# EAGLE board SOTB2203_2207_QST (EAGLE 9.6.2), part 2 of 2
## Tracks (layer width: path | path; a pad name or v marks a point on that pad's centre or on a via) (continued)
PKG1/FR_CO_CH4/FR_CI_CH3  (via drill 0.3) (continued)
  Top 0.152: PKG1.71 58.83,77.28 59.24,76.87 66.99,76.87 73.13,83.01 73.13,112.99 66.99,119.13 65.01,119.13 v64.68,119.46 | v64.71,118.25 64.67,118.22 PKG1.121
  Bottom 0.152: v64.71,118.25 64.68,118.27 v64.68,119.46
PKG1/FR_SO  (via drill 0.3)
  Top 0.152: PKG1.113 v71.4,106.12 v71.41,106.12 | v73.74,106.12 74.34,106.72 74.34,107.66 73.69,108.31 73.69,113.22 67.22,119.69 65.82,119.69 65.16,120.34 64.31,120.34 64.22,120.25 36.53,120.25 29.75,113.47 29.75,98.87 29.1,98.22 29.1,97.48 29.47,97.11 29.47,92.98 28.82,92.33 28.82,91.59 29.19,91.22 29.19,65.39 29.1,65.3 29.1,63.27 29.72,62.65 29.72,35.38 37.02,28.07 66.93,28.07 67.26,27.75 v67.26,27.19 | v67.26,25.14 67.38,25.02 67.38,18.97 68.5,17.85 CN1.A19 69.93,16.57 69.93,6.24 CN5.A19
  Bottom 0.152: v71.41,106.12 v73.74,106.12 | v67.26,27.19 v67.26,25.14
PKG1/FR_SO_CH1/FR_SI_CH2  (via drill 0.3)
  Top 0.152: PKG1.153 43.88,118.16 43.18,118.85 37.12,118.85 31.15,112.88 31.15,97.33 30.59,96.77 30.59,91.59 30.03,91.03 30.03,82.66 36.66,76.03 40.29,76.03 v40.62,75.7 | PKG1.43 40.62,78.43 v40.66,78.4
  Bottom 0.152: v40.66,78.4 40.62,78.36 v40.62,75.7
PKG1/FR_SO_CH2/FR_SI_CH3  (via drill 0.3)
  Top 0.152: v74.3,86.62 73.97,86.29 73.97,82.66 67.34,76.03 58.89,76.03 58.34,76.59 53.25,76.59 52.69,77.15 37.12,77.15 31.15,83.12 31.15,89.32 31.7,89.88 PKG1.33 | PKG1.83 71.42,86.62 v71.82,87.02
  Bottom 0.152: v74.3,86.62 74.29,86.63 72.25,86.63 71.86,87.02 v71.82,87.02
PKG1/FR_SO_CH3/FR_SI_CH4  (via drill 0.3)
  Top 0.152: PKG1.73 60.12,77.55 60.52,77.15 66.88,77.15 72.85,83.12 72.85,112.88 66.88,118.85 63.45,118.85 v63.37,118.93 | PKG1.123 63.38,117.54 v63.34,117.57
  Bottom 0.152: v63.37,118.93 63.37,117.59 v63.34,117.57
PKG1/TFT_CO  (via drill 0.3)
  Top 0.152: PKG1.149 46.48,117.94 v46.81,118.28 | v46.81,120.85 46.48,120.53 36.41,120.53 29.47,113.59 29.47,98.98 28.82,98.33 28.82,97.37 29.19,97 29.19,93.09 28.54,92.44 28.54,91.48 28.91,91.11 28.91,65.51 28.82,65.41 28.82,63.15 29.44,62.53 29.44,35.26 36.91,27.79 65.66,27.79 65.99,27.47 v65.99,27.19 | v65.99,25.14 66.01,25.12 66.01,23.03 CN1.C20
  Route15 0.152: CN1.C20 64.81,21.63 64.81,11.34 CN5.C20
  Bottom 0.152: v46.81,118.28 v46.81,120.85 | v65.99,27.19 v65.99,25.14
PKG1/TFT_CO_CH2/TFT_CI_CH1  (via drill 0.3)
  Top 0.152: PKG1.29 32.23,92.47 31.75,92.96 v31.75,95.12 | PKG1.142 51.02,118.56 50.41,119.16 44.73,119.16 44.2,119.69 36.76,119.69 30.31,113.24 30.31,98.18 v29.98,97.85
  Bottom 0.152: v31.75,95.12 31.75,97.52 31.42,97.85 v29.98,97.85
PKG1/TFT_CO_CH3/TFT_CI_CH2  (via drill 0.3)
  Top 0.152: PKG1.22 31.24,97.03 30.87,96.65 30.87,91.48 30.31,90.92 30.31,82.78 36.78,76.31 51.63,76.31 52.35,76.31 52.9,75.75 56.82,75.75 v57.15,75.42 | PKG1.69 57.52,78.11 57.19,77.78 v57.19,77.75
  Bottom 0.152: v57.19,77.75 57.19,75.46 v57.15,75.42
PKG1/TFT_CO_CH4/TFT_CI_CH3  (via drill 0.3)
  Top 0.152: PKG1.62 52.98,77.26 53.37,76.87 58.45,76.87 59.01,76.31 67.22,76.31 73.69,82.78 73.69,102.92 v74.02,103.25 | PKG1.109 71.41,103.53 v71.69,103.25
  Bottom 0.152: v74.02,103.25 v71.69,103.25
PKG1/TFT_SO  (via drill 0.3)
  Top 0.152: PKG1.104 71.97,100.28 72.29,100.59 72.29,108 72.13,108.16 v71.97,108.16 | v73.74,107.41 73.41,107.74 73.41,113.11 67.11,119.41 65.7,119.41 65.05,120.06 64.43,120.06 64.34,119.97 36.65,119.97 30.03,113.35 30.03,98.75 29.38,98.1 29.38,97.6 29.75,97.23 29.75,92.86 29.1,92.21 29.1,91.71 29.47,91.34 29.47,65.28 29.38,65.18 29.38,63.38 30,62.77 30,35.49 37.14,28.35 68.22,28.35 68.57,28.01 v68.57,27.19 | CN1.C19 68.57,23.01 v68.57,25.14
  Route15 0.152: CN1.C19 68.34,22.93 67.4,21.99 67.4,11.29 CN5.C19
  Bottom 0.152: v71.97,108.16 71.97,107.56 72.12,107.41 v73.74,107.41 | v68.57,27.19 v68.57,25.14
PKG1/TFT_SO_CH1/TFT_SI_CH2  (via drill 0.3)
  Top 0.152: PKG1.30 31.8,91.83 v31.75,91.78 | v29.7,91.96 30.03,92.29 30.03,97 30.59,97.56 30.59,113.12 36.88,119.41 44.08,119.41 44.61,118.88 49.3,118.88 49.73,118.45 PKG1.144 | v29.7,91.96
  Bottom 0.152: v29.7,91.96 31.57,91.96 v31.75,91.78
PKG1/TFT_SO_CH2/TFT_SI_CH3  (via drill 0.3)
  Top 0.152: PKG1.24 31.47,95.72 31.15,95.4 31.15,91.36 31.13,91.35 31.12,91.33 30.59,90.8 30.59,82.89 36.89,76.59 52.46,76.59 53.02,76.03 57.74,76.03 57.97,75.8 v57.97,75.7 | PKG1.70 v58.17,77.76 v58.17,77.75
  Bottom 0.152: v58.17,77.75 57.97,77.55 v57.97,75.7
PKG1/TFT_SO_CH3/TFT_SI_CH4  (via drill 0.3)
  Top 0.152: PKG1.64 54.27,77.5 54.63,77.15 58.57,77.15 59.13,76.59 67.11,76.59 73.41,82.89 73.41,103.85 v73.74,104.18 | v71.69,104.18 PKG1.110
  Bottom 0.152: v73.74,104.18 v71.69,104.18
PKG4/A_SOUT_CH1  (via drill 0.3)
  Top 0.152: PKG4.15 114.18,48.39 v117.54,48.39 | CN7.A20 85.16,143.77 85.16,133.42 CN3.A20 82.64,130.9 82.64,123.26 83.97,121.93 114.16,121.93 122.03,114.06 122.03,72.84 122.48,72.39 122.48,59.47 123.14,58.82 123.14,55.84 122.48,55.19 122.48,48.55 v122.31,48.38
  Bottom 0.152: v117.54,48.39 122.3,48.39 v122.31,48.38
PKG4/A_SOUT_CH2  (via drill 0.3)
  Top 0.152: v101.77,71.82 101.58,71.62 PKG4.55 | v101.78,74.3 102.11,73.97 108.2,73.97 109.13,74.9 110.15,74.9 110.43,75.18 117.22,75.18 117.36,75.04 117.36,72.73 v118.81,71.29 | CN7.A19 82.62,143.77 82.62,133.42 CN3.A19 80.12,130.92 80.12,122.52 81.27,121.37 113.93,121.37 121.47,113.83 v121.47,72.15
  Bottom 0.152: v101.77,71.82 101.77,74.29 v101.78,74.3 | v118.81,71.29 120.61,71.29 v121.47,72.15
PKG4/A_SOUT_CH3  (via drill 0.3)
  Top 0.152: v75.7,53.53 75.7,55.57 76.03,55.89 76.03,62.02 74.82,63.23 74.82,64.93 75.47,65.58 75.47,82.3 75.74,82.57 75.74,86.82 75.46,87.1 75.46,107.84 75.64,108.02 75.64,112.47 72.46,115.64 72.46,130.88 CN3.A16 75,133.42 75,143.77 CN7.A16 | v78.18,55.8 78.96,55.8 79.19,55.58 PKG4.95
  Bottom 0.152: v75.7,53.53 75.7,53.47 76.02,53.16 76.28,53.16 77.15,54.03 77.15,54.76 v78.18,55.8
PKG4/A_SOUT_CH4  (via drill 0.3)
  Top 0.152: PKG4.135 94.39,35.82 v94.39,32.43 | CN3.C19 81.35,122.88 82.24,121.99 82.3,121.93 82.58,121.65 114.05,121.65 121.75,113.94 121.75,72.73 122.21,72.27 122.21,59.36 122.86,58.71 122.86,55.95 122.21,55.3 122.21,52.07 121.65,51.52 121.65,42.79 122.86,41.58 122.86,38.26 122.21,37.61 122.21,35.72 114.28,27.79 105.86,27.79 105.13,27.06 104.39,27.06 104.07,27.39 102.14,27.39 101.49,28.04 95.79,28.04 95.44,27.69 v94.65,27.69
  Route15 0.152: CN7.C19 82.62,138.69 82.62,128.34 CN3.C19
  Bottom 0.152: v94.39,32.43 94.39,27.94 v94.65,27.69
PKG4/FR_CO  (via drill 0.3)
  Top 0.152: PKG4.1 v118.24,39.33 v118.25,39.32 | v120.3,39.32 119.97,38.99 119.97,36.65 113.35,30.03 105.69,30.03 105.16,30.56 87.11,30.56 86.49,29.94 85.05,29.94 84.4,30.59 78.05,30.59 77.4,29.94 v77.4,27.19 | v77.4,25.14 77.55,24.99 77.55,19.25 78.81,17.99 CN1.A15 80.09,16.57 80.09,6.42 80.09,6.24 CN5.A15
  Bottom 0.152: v118.25,39.32 v120.3,39.32 | v77.4,27.19 v77.4,25.14
PKG4/FR_CO_CH2/FR_CI_CH1  (via drill 0.3)
  Top 0.152: PKG4.151 104.83,32.08 106.03,30.87 113.01,30.87 119.13,36.99 119.13,52.56 119.69,53.12 119.69,58.29 120.25,58.85 120.25,67.45 113.45,74.25 111.01,74.25 v110.68,74.58 | PKG4.41 v110.67,72.24 v110.68,72.25
  Bottom 0.152: v110.68,72.25 v110.68,74.58
PKG4/FR_CO_CH3/FR_CI_CH2  (via drill 0.3)
  Top 0.152: PKG4.81 v77.76,64.67 v77.75,64.68 | v75.42,64.68 75.75,65.01 75.75,67.45 82.55,74.25 91.22,74.25 91.78,73.69 96.86,73.69 97.42,73.13 98,73.13 98.08,73.13 112.99,73.13 119.13,66.99 119.13,59.31 118.65,58.83 PKG4.31
  Bottom 0.152: v77.75,64.68 v75.42,64.68
PKG4/FR_CO_CH4/FR_CI_CH3  (via drill 0.3)
  Top 0.152: PKG4.121 85.33,32.05 85.29,32.01 v85.29,31.75 | PKG4.71 91.17,72.72 90.76,73.13 83.01,73.13 76.87,66.99 76.87,37.01 83.01,30.87 84.97,30.87 v85.3,30.54
  Bottom 0.152: v85.29,31.75 v85.3,31.75 v85.3,30.54
PKG4/FR_SO  (via drill 0.3)
  Top 0.152: PKG4.113 v78.6,43.88 v78.59,43.87 | v76.26,43.87 76.26,43.02 75.66,42.41 75.66,41.91 75.75,41.82 75.75,27.96 v74.98,27.19 | v74.98,25.14 74.98,19.21 76.27,17.92 CN1.A16 77.53,16.59 77.53,6.42 77.53,6.22 CN5.A16
  Bottom 0.152: v78.59,43.87 v76.26,43.87 | v74.98,27.19 v74.98,25.14
PKG4/FR_SO_CH1/FR_SI_CH2  (via drill 0.3)
  Top 0.152: PKG4.153 106.12,31.84 106.82,31.15 112.88,31.15 118.85,37.12 118.85,52.67 119.41,53.23 119.41,58.41 119.97,58.97 119.97,67.34 113.34,73.97 109.71,73.97 v109.38,74.3 | PKG4.43 109.38,71.57 v109.13,71.82
  Bottom 0.152: v109.13,71.82 109.38,72.06 v109.38,74.3
PKG4/FR_SO_CH2/FR_SI_CH3  (via drill 0.3)
  Top 0.152: v75.7,63.38 76.03,63.71 76.03,67.34 82.66,73.97 91.11,73.97 91.66,73.41 96.75,73.41 97.31,72.85 112.88,72.85 118.85,66.88 118.85,60.68 118.3,60.12 PKG4.33 | PKG4.83 78.58,63.38 v78.18,62.98
  Bottom 0.152: v75.7,63.38 75.71,63.37 77.75,63.37 78.14,62.98 v78.18,62.98
PKG4/FR_SO_CH3/FR_SI_CH4  (via drill 0.3)
  Top 0.152: PKG4.73 89.88,72.45 89.48,72.85 83.12,72.85 77.15,66.88 77.15,37.12 83.12,31.15 86.69,31.15 v86.77,31.07 | PKG4.123 86.62,32.46 v86.66,32.43
  Bottom 0.152: v86.66,32.43 86.66,31.18 v86.77,31.07
PKG4/TFT_CO  (via drill 0.3)
  Top 0.152: PKG4.149 103.53,31.88 103.36,31.72 v103.2,31.72 | v103.2,29.95 102.87,30.28 87.23,30.28 86.61,29.66 84.93,29.66 84.28,30.31 79.18,30.31 78.71,29.84 v78.71,27.19 | v78.71,25.14 78.78,25.07 78.78,22.96 CN1.C15
  Route15 0.152: CN1.C15 77.55,21.67 77.55,11.5 77.55,11.3 CN5.C15
  Bottom 0.152: v103.2,31.72 v103.2,29.95 | v78.71,27.19 v78.71,25.14
PKG4/TFT_CO_CH2/TFT_CI_CH1  (via drill 0.3)
  Top 0.152: PKG4.29 117.77,57.52 118.06,57.23 v118.25,57.23 | v120.58,56.9 120.25,56.57 120.25,52.88 119.69,52.33 119.69,36.76 113.24,30.31 105.8,30.31 105.27,30.84 99.59,30.84 98.97,31.45 PKG4.142
  Bottom 0.152: v118.25,57.23 118.58,56.9 v120.58,56.9
PKG4/TFT_CO_CH3/TFT_CI_CH2  (via drill 0.3)
  Top 0.152: PKG4.22 118.76,52.98 119.13,53.35 119.13,58.52 119.69,59.08 119.69,67.22 113.22,73.69 97.65,73.69 97.1,74.25 92.51,74.25 v92.18,74.58 | PKG4.69 92.47,71.89 92.81,72.22 v92.81,72.25
  Bottom 0.152: v92.18,74.58 92.81,73.95 v92.81,72.25
PKG4/TFT_CO_CH4/TFT_CI_CH3  (via drill 0.3)
  Top 0.152: PKG4.62 97.03,72.74 96.63,73.13 91.55,73.13 90.99,73.69 82.78,73.69 76.31,67.22 76.31,47.08 v75.98,46.75 | PKG4.109 78.59,46.48 v78.31,46.75
  Bottom 0.152: v75.98,46.75 v78.31,46.75
PKG4/TFT_SO  (via drill 0.3)
  Top 0.152: PKG4.104 78.03,49.73 77.71,49.4 77.71,42.49 v78.03,42.16 | v76.26,42.16 76.59,41.83 76.59,27.61 v76.17,27.19 | CN1.C16 76.17,23.03 v76.17,25.14
  Route15 0.152: CN1.C16 75.01,21.67 75.01,11.5 75.01,11.3 CN5.C16
  Bottom 0.152: v78.03,42.16 v76.26,42.16 | v76.17,27.19 v76.17,25.14
PKG4/TFT_SO_CH1/TFT_SI_CH2  (via drill 0.3)
  Top 0.152: PKG4.30 118.2,58.17 v118.25,58.22 | v120.3,58.04 119.97,57.71 119.97,53 119.41,52.44 119.41,36.88 113.12,30.59 105.92,30.59 105.39,31.12 100.7,31.12 100.28,31.55 PKG4.144
  Bottom 0.152: v120.3,58.04 118.43,58.04 v118.25,58.22
PKG4/TFT_SO_CH2/TFT_SI_CH3  (via drill 0.3)
  Top 0.152: PKG4.24 118.53,54.27 118.85,54.6 118.85,58.64 118.87,58.65 118.88,58.67 119.41,59.2 119.41,67.11 113.11,73.41 97.54,73.41 96.98,73.97 91.89,73.97 91.01,74.86 v90.95,74.86 | PKG4.70 v91.83,72.24 v91.83,72.25
  Bottom 0.152: v91.83,72.25 91.83,73.98 v90.95,74.86
PKG4/TFT_SO_CH3/TFT_SI_CH4  (via drill 0.3)
  Top 0.152: PKG4.64 95.72,72.5 95.37,72.85 91.43,72.85 90.87,73.41 82.89,73.41 76.59,67.11 76.59,46.15 v76.26,45.82 | v78.31,45.82 PKG4.110
  Bottom 0.152: v76.26,45.82 v78.31,45.82
TFT_CI  (via drill 0.3, 0.35)
  Top 0.152: PKG4.102 77.81,51.02 77.43,50.64 77.43,39.65 77.82,39.25 79.28,39.25 84.3,34.22 v84.62,34.22 | PKG1.102 72.19,98.97 72.57,99.36 72.57,110.28 72.14,110.71 70.63,110.71 65.56,115.78 v65.38,115.78 | v65.38,121.23 65.05,120.9 64.08,120.9 63.99,120.81 48.2,120.81 47.27,121.74 46.44,121.74 45.79,121.09 36.18,121.09 28.91,113.82 28.91,112.02 27.98,111.09 27.98,110.3 28.63,109.65 28.63,99.33 27.98,98.68 27.98,97.02 28.35,96.65 28.35,93.44 27.7,92.79 27.7,91.13 28.07,90.76 28.07,78.33 27.42,77.68 27.42,76.53 v27.75,76.2 28.07,75.87 28.07,67.04 27.42,66.39 27.42,65.89 27.66,65.65 v27.66,65.38 27.98,65.05 27.98,62.81 28.6,62.19 28.6,34.91 36.56,26.96 63.67,26.96 64.32,26.3 84.11,26.3 84.76,25.65 85.37,25.65 v85.69,25.98 86.02,26.3 86.02,27.88 86.4,28.26 87.19,28.26 87.81,28.88 101.84,28.88 102.49,28.23 103.91,28.23 104.32,28.63 113.93,28.63 121.37,36.07 121.37,37.95 122.02,38.61 122.02,40.03 121.09,40.97 121.09,51.75 121.65,52.31 121.65,55.53 122.3,56.19 122.3,58.47 121.65,59.13 121.65,68.03 120.53,69.15 120.53,76.3 119.55,77.28 v119.55,78.89 | CN4.C17 23,76.2 v25.65,76.2 | v59.4,34.3 58.9,34.3 58.48,34.72 38.88,34.72 34.72,38.88 34.72,44.28 v34.3,44.7 34.3,44.9 34.72,45.32 34.72,65.72 v35,66 v37.7,68.7 38.28,69.28 65.82,69.28 69.5,65.6 69.5,61.5 67.5,59.5 JP2.3 | JP14.3 113.5,105.5 115.5,107.5 115.5,111.6 111.82,115.28 84.28,115.28 v83.7,114.7 80.72,111.72 80.72,91.32 80.3,90.9 v80.3,90.3 80.3,89.9 80.72,89.48 80.72,84.88 84.88,80.72 104.48,80.72 104.9,80.3 v105.4,80.3 106.05,79.65 116.95,79.65 v117.6,79
  Route2 0.152: v27.66,65.38 34,65.38 34.62,66 v35,66
  Route15 0.152: CN4.C17 21.69,77.51 11.28,77.51 CN8.C17
  Bottom 0.152: v65.38,115.78 v65.38,121.23 | v27.75,76.2 v25.65,76.2 | v84.62,34.22 84.62,29.09 85.69,28.01 v85.69,25.98 | v59.4,34.3 59.5,34.4 JP4.3 | v34.3,44.7 34.5,44.5 JP6.3 | v37.7,68.7 43.8,68.7 44.5,68 JP8.3 | v105.4,80.3 105.5,80.4 JP16.3 | v80.3,90.3 80.5,90.5 JP10.3 | v83.7,114.7 89.8,114.7 90.5,114 JP12.3 | v117.6,79 119.44,79 v119.55,78.89
TFT_SI  (via drill 0.3, 0.35)
  Top 0.152: PKG1.150 45.83,118.23 v45.78,118.28 | v104.3,31.72 104.17,31.84 PKG4.150 | v45.54,121.69 45.22,121.37 36.07,121.37 28.63,113.93 28.63,112.13 27.7,111.2 27.7,110.19 28.35,109.54 28.35,99.45 27.7,98.8 27.7,96.91 28.07,96.53 28.07,93.56 27.42,92.91 27.42,91.02 27.79,90.64 27.79,78.45 27.14,77.8 27.14,75.34 v27.47,75.01 27.79,74.68 27.79,67.16 27.05,66.41 27.05,65.13 27.7,64.48 27.7,62.69 28.32,62.07 28.32,46.32 27.94,45.94 v27.94,45.39 28.32,45.01 28.32,34.8 36.44,26.68 36.5,26.68 63.55,26.68 64.2,26.02 83.99,26.02 84.65,25.37 85.95,25.37 86.3,25.73 86.3,27.77 86.51,27.98 87.3,27.98 87.92,28.6 101.72,28.6 102.37,27.95 v104.76,27.95 105.16,28.35 114.05,28.35 121.65,35.95 121.65,37.84 122.3,38.49 122.3,40.15 121.37,41.08 121.37,51.63 121.93,52.19 121.93,55.42 122.58,56.07 122.58,58.59 121.93,59.24 121.93,68.15 120.81,69.27 120.81,76.42 120.2,77.03 v120.2,79.8 | v25.65,75 18.84,75 17.85,74.01 CN4.A16 16.6,72.48 6.21,72.48 CN8.A16 | JP7.1 35.08,54.42 | 35.08,54.42 35,54.5 | 35,54.5 35,65 39,69 54,69 54.42,68.58 JP1.1 | 35,54.5 35,54.34 | 35,54.34 35,47.1 | 35,47.1 35,47 | 35,47 35,46.9 | 35,46.9 35,39 39,35 49.33,35 | 49.58,35.08 49.58,35.25 | JP5.1 49.58,35.25 | 49.33,35 49.83,35 | 49.83,35 65.5,35 69,38.5 69,49 68.42,49.58 JP3.1 | 35,54.34 35.08,54.42 | v35.7,46.2 35.7,46.8 35.5,47 35.1,47 | 35,47 35.1,47 | 35,47.1 35.1,47 | 35.1,47 35,46.9 | JP11.1 81.08,100.42 | 81.08,100.42 81,100.5 | 81,100.5 81,111 85,115 100,115 100.42,114.58 JP13.1 | 81,100.5 81,100.34 | 81,100.34 81,85 85,81 95.41,81 | 95.58,81.08 95.58,81.17 | 95.58,81.17 JP9.1 | 95.41,81 95.75,81 | 95.75,81 v110.2,81 111.5,81 115,84.5 115,95 114.42,95.58 JP15.1
  Top 0.152: 81,100.34 81.08,100.42 | 49.58,35.25 49.33,35 | 95.75,81 95.58,81.17 | 95.58,81.17 95.41,81 | 49.58,35.25 49.83,35
  Bottom 0.152: v45.54,121.69 45.78,121.45 v45.78,118.28 | v104.76,27.95 104.76,31.26 v104.3,31.72 | v27.47,75.01 v25.66,75.01 v25.65,75 | v27.94,45.39 34.9,45.39 v35.7,46.2 | v110.2,81 111,80.2 119.8,80.2 v120.2,79.8
VBN  (via drill 0.3, 0.35, 0.8, 1.27)
  Top 0.305: PKG1.158 40.62,111.97 v40.5,111.84 | PKG1.118 66.03,109.38 v65.89,109.51 | PKG1.38 37.95,86.62 v38.07,86.5 | PKG1.78 63.38,83.89 v63.5,84.01 | PKG4.78 86.62,66.08 v86.5,65.95 | PKG4.38 112.13,63.38 v112.01,63.5 | PKG4.158 109.38,37.97 v109.47,38.06 | PKG4.118 83.88,40.62 v84,40.5
  Top 0.508: CN4.C21 21.66,87.7 11.31,87.7 CN8.C21
  Route2 0.305: v95.29,39.46 95.29,37.85 95.89,37.25 108.66,37.25 v109.47,38.06 | v112.01,63.5 112.51,63.5 112.85,63.84 112.85,77.24 111.91,78.17 v109.92,78.17 | v65.7,77.75 63.86,77.75 63.5,78.11 v63.5,84.01 | v38.3,77.75 38.3,75.04 38.71,74.63 39.33,74.63 44.67,69.28 47.7,69.28 49.58,67.4 JP8.5 | v49.39,106.27 51.4,106.27 52.42,107.29 64.65,107.29 65.13,107.77 65.13,109.13 65.51,109.51 v65.89,109.51
  Route2 1.016: v71.47,78.01 72.84,76.64 72.84,70.23 v73.62,69.45
  Bottom 0.305: v40.5,111.84 C20.1 | v65.89,109.51 C15.1 | v38.07,86.5 C5.1 | v63.5,84.01 C10.1 | v86.5,65.95 C70.1 | v112.01,63.5 C65.1 | v109.47,38.06 109.5,38.09 C80.1 | v84,40.5 C75.1 | JP8.5 48.5,65.42 C35.1 49.38,60 v55,60 | JP2.5 65.42,55.5 v62.5,55.5 C30.1 | JP4.5 55.5,38.58 v55.5,41.5 C25.1 | JP6.5 38.58,48.5 C40.1 44.62,50 v56,50 | JP10.5 84.6,94.48 89.11,94.48 C50.1 90.62,96 v102,96 | JP12.5 94.5,111.42 C45.1 95.38,106 v101,106 | JP14.5 111.42,101.5 v108.5,101.5 C60.1 | JP16.5 101.5,84.58 v101.5,87.5 C55.1
  Bottom 1.27: v32.5,77.5 32.5,82.37 31.25,83.62 29.57,83.62 28.9,84.29 U$8.+ 22.95,86.41 CN4.C21
  other vias: 83,67 84,68 82,66
  pour Route15: 55,70 54,69 54,35 55,34 65,34 70,39 70,65 65,70
  pour Route15: 32,79 111,79 111,77 110,76 32,76 31,77 31,78
  pour Route15: 39,116 34,111 34,80 33,79 51,79 50,80 50,115 49,116
  pour Route15: 85,70 80,65 80,39 85,34 95,34 96,35 96,69 95,70
  pour Route15: 101,116 100,115 100,80 99,79 111,79 116,84 116,111 111,116
  pour Route15: 65,70 65,65 85,65 85,70
VBP  (via drill 0.3, 0.35, 0.8, 1.27)
  Top 0.305: PKG1.157 41.27,112.03 41.44,111.86 v42,111.86 | PKG1.117 66.14,108.72 65.92,108.51 v65.92,108 | PKG1.37 37.91,87.28 38.04,87.41 v38.04,88 | v61.99,84 62.51,84 62.73,83.78 PKG1.77 | v88,65.95 87.43,65.95 87.28,66.11 PKG4.77 | v112.03,62.01 112.03,62.49 112.27,62.73 PKG4.37 | v108,38.07 108.5,38.07 108.72,37.84 PKG4.157 | PKG4.117 83.77,41.27 83.97,41.48 v83.97,42
  Top 0.508: CN4.C12 21.7,62.34 11.27,62.34 CN8.C12
  Route2 0.305: v83.97,42 97.57,42 97.96,42.39 97.96,43.74 98.14,43.92 v100.66,43.92 | v88,65.95 v88,71.54 | v38.04,88 37.28,87.24 37.28,73.35 v38.17,72.46 | v42,111.86 42.73,112.59 54.66,112.59 54.92,112.33 54.92,111.2 v55.05,111.08 | v107.96,71.82 108.65,72.5 108.65,78.49 106.03,81.11 103.17,81.11 102.96,81.33 JP16.4
  Route2 1.016: v78.41,72.04 77.16,73.29 77.16,79.77 v76.38,80.55
  Bottom 0.305: v42,111.86 C19.1 | v65.92,108 C14.1 | v38.04,88 C4.1 | v61.99,84 C9.1 | v88,65.95 C69.1 | v112.03,62.01 v112.02,62 C64.1 | v108,38.07 C79.1 | v83.97,42 C74.1 | JP6.4 38.04,46.5 v41.5,46.5 C39.1 | JP4.4 57.5,38.04 C24.1 56.5,44.12 56.5,47 55.5,48 50,48 49.5,48.5 v49,48.5 | JP2.4 65.96,57.5 C29.1 59.88,56.5 56.5,56.5 56,56 v48,56 | JP8.4 46.5,65.96 v46.5,62.5 C34.1 | JP10.4 84.04,92.5 v87.5,92.5 C49.1 | JP12.4 92.5,111.96 v92.5,108.5 C44.1 | JP14.4 111.96,103.5 C59.1 105.88,102.5 102.5,102.5 102,102 v94,102 | JP16.4 103.5,84.04 C54.1 102.5,90.12 102.5,93 101.5,94 96,94 95.5,94.5 v95,94.5
  Bottom 1.27: v32.5,72.5 32.5,67.61 30.93,66.04 29.86,66.04 28.9,65.08 U$7.+ 23.01,63.49 CN4.C12
  other vias: 67,83 68,84 66,82
  pour Route15: 33,71 34,70 34,39 39,34 49,34 50,35 50,70 51,71
  pour Route15: 32,74 110,74 111,73 111,71 32,71 31,72 31,73
  pour Route15: 55,116 54,115 54,81 55,80 65,80 70,85 70,111 65,116
  pour Route15: 85,116 80,111 80,85 85,80 95,80 96,81 96,115 95,116
  pour Route15: 99,71 100,70 100,35 101,34 111,34 116,39 116,66 111,71
  pour Route15: 65,85 65,80 85,80 85,85
VCCQ  (via drill 0.3, 0.35, 1.27)
  Top 0.305: PKG1.159 39.98,112.35 39.47,111.85 v39,111.85 39,111.39 39.23,111.16 48.68,111.16 49.84,112.32 51.36,112.32 51.67,112.64 PKG1.141 51.67,117.12 v51.66,117.13 | PKG1.119 66.64,110.03 65.88,110.78 v65.88,111 65.4,111 65.21,110.81 65.21,101.28 66.32,100.17 66.32,98.64 66.64,98.33 PKG1.101 | PKG1.39 37.36,85.97 38.13,85.21 v38.13,84.99 38.75,85.61 v38.75,93.62 38.75,94.75 37.68,95.82 37.68,97.36 37.36,97.67 PKG1.21 | PKG1.79 64.03,83.36 64.75,84.09 v65.02,84.09 65.02,84.65 64.82,84.85 v57.12,84.85 55.79,84.85 54.62,83.68 52.64,83.68 52.33,83.36 PKG1.61 | PKG4.79 85.97,66.48 85.42,65.93 v85.01,65.93 | v85.01,65.93 v85,65.93 | PKG4.61 97.67,66.26 97.43,66.01 96.88,66.01 96.6,65.73 95.39,65.73 94.83,65.18 v92.96,65.18 85.27,65.18 85.01,65.44 v85.01,65.93 | PKG4.39 112.64,64.03 111.99,64.67 v111.99,65 111.55,65 111.24,64.69 v111.24,56.67 111.24,55.29 112.32,54.21 112.32,52.55 112.55,52.33 PKG4.21 | PKG4.159 110.03,37.66 110.41,38.04 v111.01,38.04 111.01,38.57 110.78,38.8 101.39,38.8 100.27,37.68 98.64,37.68 98.33,37.36 PKG4.141 | PKG4.119 83.36,39.98 84.04,39.3 84.04,39.02 | v84.04,39 84.04,39.02 | PKG4.101 83.45,51.67 83.68,51.45 83.68,49.84 84.71,48.81 84.71,39.18 84.55,39.02 84.04,39.02
  Top 2.54: CN4.A1 CN4.B1 CN4.C1
  Route2 0.305: v84.04,39 82.16,39 81.83,38.67 v81.83,31.19 | v111.7,31.75 111.7,37.59 111.25,38.04 v111.01,38.04 | v92.96,65.18 92.39,65.18 92.34,65.23 91.74,65.23 91.31,64.8 91.31,59.81 91.79,59.33 93.9,59.33 94.21,59.02 v94.21,57.41 | v103.35,56.03 110.6,56.03 v111.24,56.67 | v57.12,84.85 57.59,84.85 57.64,84.8 58.25,84.8 58.67,85.23 58.67,90.38 58.46,90.59 56.1,90.59 55.78,90.91 v55.78,92.5 | v38.75,93.62 39.22,94.09 v46.6,94.09 | v65.88,111 62.1,111 61.7,111.4 61.7,117.46 v61.81,117.57
  Route15 2.54: CN4.A1 CN8.C1 CN8.B1 CN8.A1
  Bottom 0.305: v39,111.85 C18.1 | v65.88,111 C13.1 | v38.13,84.99 C3.1 | v65.02,84.09 65.02,85.11 C8.1 | v85,65.93 C68.1 | v111.99,65 C63.1 | v111.01,38.04 C78.1 | v84.04,39 C73.1 | JP7.4 43.34,62.04 C33.1 45.5,59.88 45.5,56 46,55.5 v46.5,55.5 | JP1.4 62.04,60.66 C28.1 59.88,58.5 56,58.5 55.5,58 v55.5,57.5 | JP3.4 60.66,41.96 C23.1 58.5,44.12 58.5,48 58,48.5 v57.5,48.5 | JP5.4 41.96,43.34 C38.1 43.12,44.62 44,45.5 48,45.5 48.5,46 v48.5,46.5 | JP9.4 87.96,89.34 C48.1 90.12,91.5 94,91.5 94.5,92 v94.5,92.5 | JP11.4 89.34,108.04 C43.1 91.5,105.88 91.5,102 92,101.5 v92.5,101.5 | JP13.4 108.04,106.66 C58.1 105.88,104.5 102,104.5 101.5,104 v101.5,103.5 | JP15.4 106.66,87.96 C53.1 104.5,90.12 104.5,94 104,94.5 v103.5,94.5
  Bottom 1.27: U$6.+ 27.11,35.61 | 27.11,35.61 26,35.61 | 26,35.61 24.89,35.61 | 24.89,35.61 22.95,35.61 CN4.C1 | v29.5,28 27,28 26,29 26,34.5 | 26,34.5 26,35.61 | 26,34.5 24.89,35.61 | 26,34.5 27.11,35.61
  other vias: 97,57 99,57 97,55 99,55 97,53 99,53 97,47 99,47 97,49 99,49 97,51 99,51 51,103 53,103 51,101 53,101 51,99 53,99 51,93 53,93 51,95 53,95 51,97 53,97 51,57 53,57 51,55 53,55 51,53 53,53 51,47 53,47 51,49 53,49 51,51 53,51 97,103 99,103 97,101 99,101 97,99 99,99 97,93 99,93 97,95 99,95 97,97 99,97
  pour Top: 48,104 46,102 46,94 48,92 56,92 58,94 58,102 56,104
  pour Top: 94,58 92,56 92,48 94,46 102,46 104,48 104,56 102,58
  pour Route15: 29,33.5 49.5,33.5 50.5,34.5 50.5,57.5 51,58 53,58 53.5,57.5 53.5,34.5 54.5,33.5 95.5,33.5 96.5,34.5 96.5,57.5 97,58 99,58 99.5,57.5 99.5,34.5 100.5,33.5 111.5,33.5 116.5,38.5 116.5,111.5 111.5,116.5 100.5,116.5 99.5,115.5 99.5,92.5 99,92 97,92 96.5,92.5 96.5,115.5 95.5,116.5 54.5,116.5 53.5,115.5 53.5,92.5 53,92 51,92 50.5,92.5 50.5,122 52,123.5 113,123.5 123.5,113 123.5,37 113,26.5 29,26.5 27.5,28 27.5,32
  pour Bottom (no thermals): 17,37 16.5,36.5 16.5,35 17,34.5 25,34.5 25.5,34 30,34 30.5,34.5 30.5,36.5 30,37
  pour Top: 48,58 46,56 46,48 48,46 56,46 58,48 58,56 56,58
  pour Top: 94,104 92,102 92,94 94,92 102,92 104,94 104,102 102,104
VDD  (via drill 0.3, 0.35, 1.27)
  Top 0.305: PKG4.16 117.83,49.08 118.5,48.4 118.5,40.56 117.91,39.98 PKG4.2 104.56,39.98 104.08,40.45 v104.08,41.81 | PKG4.136 95.08,32.1 94.72,31.75 86.25,31.75 85.97,32.02 PKG4.122 85.97,45.66 v85.39,46.24 | PKG4.56 100.92,71.94 101.49,72.5 109.41,72.5 110.03,71.89 PKG4.42 110.03,58.35 v110.53,57.84 | PKG4.96 78.09,54.92 77.5,55.52 77.5,63.26 78.27,64.03 PKG4.82 91.57,64.03 v92.04,64.5 | PKG1.16 32.17,100.92 31.5,101.6 31.5,109.44 32.09,110.03 PKG1.2 45.71,110.03 v46.16,110.48 | PKG1.136 54.92,117.9 55.28,118.25 63.75,118.25 64.03,117.97 PKG1.122 64.03,104.48 v64.53,103.98 | PKG1.56 49.08,78.06 48.51,77.5 40.59,77.5 39.98,78.11 PKG1.42 39.98,91.81 v39.43,92.35 | PKG1.96 71.91,95.08 72.5,94.48 72.5,86.74 71.73,85.97 PKG1.82 58.39,85.97 v57.94,85.53 | 43.25,112.09 42.75,112.09 42.58,112.27 PKG1.155 42.58,115.97 42.33,116.22 42.16,116.22 41.92,115.98 PKG1.156 | 43.25,112.09 v43.49,111.85 | 43.25,112.09 44.37,112.09 44.52,112.25 PKG1.152 | PKG1.145 49.08,116.12 48.9,116.3 48.02,116.3 | 47.77,116.06 PKG1.147 | 48.02,116.3 47.77,116.06 | v45.02,111.86 46.94,111.86 47.12,112.05 PKG1.148 47.12,116.12 47.31,116.3 47.57,116.3 | 48.02,116.3 47.57,116.3 | 47.77,116.06 47.57,116.26 47.57,116.3 | PKG1.112 66.41,105.47 66.16,105.73 66.16,106.49 | PKG1.116 70.08,108.08 70.2,107.95 70.2,107.55 70.08,107.42 PKG1.115 66.41,107.42 66.16,107.17 66.16,106.49 | v65.91,106.5 66.15,106.5 66.16,106.49 | 70.3,102.42 70.3,102.72 70.14,102.88 PKG1.108 66.25,102.88 65.96,103.17 v65.96,104.99 | 70.3,102.42 70.3,102.05 | 70.3,102.05 70.3,101.11 70.11,100.92 PKG1.105 | PKG1.107 70.11,102.22
  Top 0.305: 70.11,102.22 70.12,102.22 70.3,102.05 | 70.11,102.22 70.3,102.42 | PKG1.36 33.94,87.92 33.81,88.05 33.81,88.4 33.97,88.56 35.84,88.56 PKG1.35 37.52,88.58 38.03,89.08 v38.03,89.49 38.03,90.09 37.59,90.53 PKG1.32 | PKG1.25 33.62,95.08 33.41,94.86 33.41,93.98 | 33.41,93.98 33.41,93.57 | 33.41,93.57 33.41,93.35 33.63,93.12 PKG1.28 37.7,93.12 38.04,92.79 v38.04,91 | PKG1.27 33.62,93.78 | 33.62,93.78 33.41,93.57 | 33.62,93.78 33.41,93.98 | PKG1.72 59.48,83.55 59.88,83.95 v60.52,83.95 61.02,83.95 61.42,83.55 PKG1.75 61.42,79.86 61.54,79.75 61.96,79.75 62.08,79.86 PKG1.76 | PKG1.65 54.92,79.83 55.06,79.7 56.05,79.7 | 56.05,79.7 56.38,79.7 | 56.38,79.7 56.69,79.7 56.88,79.89 PKG1.68 56.88,83.69 57.24,84.05 v58.99,84.05 | PKG1.67 56.23,79.88 | 56.23,79.88 56.05,79.7 | 56.23,79.88 56.38,79.72 56.38,79.7 | PKG4.76 87.92,70.14 88.1,70.32 88.4,70.32 88.58,70.14 PKG4.75 88.58,66.44 89.03,65.99 v89.52,65.99 90.07,65.99 90.53,66.44 PKG4.72 | 93.94,70.38 94.91,70.38 95.08,70.22 PKG4.65 | 93.94,70.38 93.6,70.38 | 93.6,70.38 93.32,70.38 93.12,70.19 PKG4.68 93.12,66.64 92.81,66.32 91.37,66.32 v91.07,66.02 | PKG4.67 93.78,70.2 | 93.78,70.2 93.6,70.38 | 93.78,70.2 93.78,70.22 93.94,70.38 | PKG4.36 116.08,62.08 116.23,61.92 116.23,61.58 116.08,61.42 PKG4.35 112.5,61.42 112.01,60.94 v112.01,60.5 112.01,59.97 112.5,59.48 PKG4.32 | 116.38,56.4 116.38,56.67 116.17,56.88 PKG4.28 114.13,56.89 112.62,56.89 112.32,57.19 112.32,58.71 111.98,59.04 v111.95,59.04 | 116.38,56.4 116.38,56.05 | 116.38,56.05 116.38,55.12 116.19,54.92 PKG4.25 | PKG4.27 116.2,56.23 | 116.2,56.23 116.38,56.4 | 116.2,56.23 116.38,56.05
  Top 0.305: PKG4.156 108.08,33.84 107.94,33.7 107.56,33.7 107.42,33.84 PKG4.155 107.42,37.47 106.87,38.02 v106.5,38.02 106.02,38.02 105.47,37.48 PKG4.152 | PKG4.145 100.92,33.85 101.12,33.66 102.05,33.66 | 102.05,33.66 102.4,33.66 | 102.4,33.66 102.65,33.66 102.88,33.88 PKG4.148 102.88,37.36 103.19,37.68 104.62,37.68 v104.98,38.04 | PKG4.147 102.22,33.84 | 102.22,33.84 102.05,33.66 | 102.22,33.84 102.4,33.66 | PKG4.116 79.81,41.92 79.63,42.11 79.63,42.4 79.81,42.58 PKG4.115 83.44,42.58 83.87,43 v83.87,43.5 83.87,44.14 83.48,44.52 PKG4.112 | PKG4.105 79.72,49.08 79.5,48.86 79.5,47.98 | 79.5,47.62 79.5,47.36 79.73,47.12 PKG4.108 83.41,47.12 83.68,46.85 83.68,45.24 v83.89,45.03 | 79.5,47.62 79.5,47.98 | PKG4.107 79.7,47.77 | 79.7,47.77 79.5,47.98 | 79.7,47.77 79.55,47.62 79.5,47.62
  Top 2.54: CN4.C32 CN4.B32 CN4.A32 CN8.C32 CN8.B32 CN8.A32
  Bottom 0.305: v43.49,111.85 v43.5,111.84 C17.1 | v45.02,111.86 45.02,110.9 C16.1 45.76,110.88 v46.16,110.48 | C12.1 v65.91,106.5 | v65.96,104.99 C11.1 64.88,104.33 v64.53,103.98 | v38.03,89.49 C2.1 | v38.04,91 C1.1 39.12,92.04 v39.43,92.35 | C7.1 60.5,83.97 v60.52,83.95 | v58.99,84.05 C6.1 58.35,85.12 v57.94,85.53 | C67.1 89.5,65.97 v89.52,65.99 | v91.07,66.02 91,65.95 C66.1 91.66,64.88 v92.04,64.5 | C62.1 v112.01,60.5 | v111.95,59.04 110.91,59.04 C61.1 110.88,58.18 v110.53,57.84 | C77.1 v106.5,38.02 | v104.98,38.04 105,38.06 C76.1 104.36,39.12 104.08,39.41 104.08,41.56 v104.08,41.81 | C72.1 v83.87,43.5 | v83.89,45.03 83.92,45 85.05,45 | 85.05,45 C71.1 | v85.39,46.24 85.05,45.9 85.05,45 | JP7.3 38.88,60.88 C31.1 C32.1 43.12,60.88 43.5,60.5 v43.5,57.5 | JP1.3 60.88,65.12 C26.1 C27.1 60.88,60.88 60.5,60.5 v57.5,60.5 | JP3.3 65.12,43.12 C21.1 C22.1 60.88,43.12 60.5,43.5 v60.5,46.5 | JP5.3 43.12,38.88 C36.1 C37.1 43.12,43.12 43.5,43.5 v46.5,43.5 | JP9.3 89.12,84.88 C46.1 C47.1 89.12,89.12 89.5,89.5 v92.5,89.5 | JP11.3 84.88,106.88 C41.1 C42.1 89.12,106.88 89.5,106.5 v89.5,103.5 | JP13.3 106.88,111.12 C56.1 C57.1 106.88,106.88 106.5,106.5 v103.5,106.5 | JP15.3 111.12,89.12 C51.1 C52.1 106.88,89.12 106.5,89.5 v106.5,92.5
  Bottom 1.27: v37.5,112.5 35.61,114.39 U$5.+ 22.95,114.39 CN4.C32
  pour Route2: 39,116 34,111 34,39 39,34 111,34 116,39 116,111 111,116
  pour Bottom (no thermals): 17,115.5 16.5,115 16.5,113.5 17,113 30,113 30.5,113.5 30.5,115 30,115.5

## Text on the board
tPlace: CN7 | CN3 | CN8 | CN4 | VDD | BOARD6 | BOARD7 | BOARD5 | BOARD8 | BOARD4 | BOARD1 | BOARD3 | BOARD2 | VCCQ | CN2 | CN6 | CN1 | CN5 | SOTB2203/2307 Board for / Heavy-ion Irradiation Test | 2024/08/18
